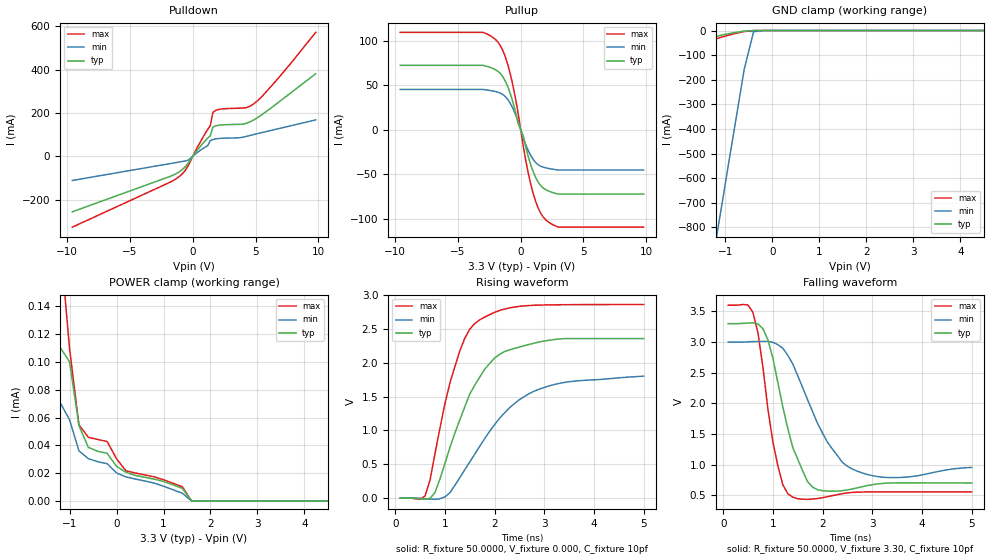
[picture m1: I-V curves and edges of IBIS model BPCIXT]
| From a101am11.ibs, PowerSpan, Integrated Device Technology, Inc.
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|   Model PCI tristate_driver
[Model]   BPCIXT
Model_type   I/O
Polarity   Non-Inverting
Enable   Active-High
Vinl = 1.16v
Vinh = 1.65v
C_comp   10.5pf   8pf   12pf
[Temperature Range]   27.0   125.0   -40.0
[Pullup Reference]   3.30V   3.00V   3.60V
[Pulldown Reference]   0.00V   0.00V   0.00V
[POWER Clamp Reference]   3.30V   3.00V   3.60V
[GND Clamp Reference]   0.00V   0.00V   0.00V
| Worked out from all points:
|   slope of the pulldown table from 0 to 0.495 V, typ, clamps not added: 13 ohm
|   slope of the pullup table from 0 to 0.495 V, typ, clamps not added: 20.4 ohm
|   GND clamp passes 1 mA (typ) near -0.47 V on its own axis
|   POWER clamp passes 1 mA (typ) near -2.20 V on its own axis
|   rising waveform, R_fixture 50.0000, V_fixture 0.000, C_fixture 10pf: 20-80 % time 802ps typ, 1.13ns min, 582ps max; typ from 0 V to 2.36 V
|   falling waveform, R_fixture 50.0000, V_fixture 3.30, C_fixture 10pf: 20-80 % time 446ps typ, 673ps min, 325ps max; typ from 3.3 V to 0.7 V
[Pulldown]
|   volt   I(typ)   I(min)   I(max)
-9.6V     -256.8mA   -112mA     -327.7mA
-1.8V     -93.12mA   -34mA      -119.8mA
-1V       -68.86mA   -26mA      -90.01mA
-400mV    -34.11mA   -19.2mA    -46.95mA
1.2V      84.05mA    49.29mA    125.1mA
1.4V      94.99mA    72.6mA     142.2mA
1.6V      134.1mA    76.97mA    201.7mA
2.2V      144.1mA    82.47mA    217.6mA
4.2V      150.9mA    90.54mA    223.7mA
5V        172.4mA    102.3mA    248.3mA
7V        256.6mA    129.6mA    372.8mA
9.8V      381.2mA    167.8mA    572.4mA
[Pullup]
|volt  I(typ)   I(min)   I(max)
-9.6V     72.37mA    45.28mA    109.5mA
-3V       72.37mA    45.28mA    109.5mA
-1.8V     65.55mA    42.08mA    98.22mA
-1.2V     53.9mA     36.95mA    80.94mA
-800mV    39.41mA    28.97mA    61.1mA
-400mV    19.13mA    16.72mA    34.19mA
400mV     -19.13mA   -16.72mA   -34.19mA
1V        -47.37mA   -33.48mA   -71.9mA
1.6V      -62.88mA   -41.03mA   -93.99mA
2.2V      -68.78mA   -43.48mA   -103.6mA
3V        -72.37mA   -45.28mA   -109.5mA
9.8V      -72.37mA   -45.28mA   -109.5mA
[GND_clamp]
|volt   I(typ)   I(min)   I(max)
-9.6V     -437.1mA   -10.59A    -530.5mA
-1.2V     -23.99mA   -851.9mA   -33.77mA
-1V       -15.53mA   -620mA     -22.63mA
-600mV    -2.506mA   -158.4mA   -4.199mA
-400mV    -152.4uA   -4.992mA   -240.4uA
-200mV    -18.8uA    -41.37uA   -20.15uA
9.8V      0A         0A         0A
[POWER_clamp]
|volt   I(typ)   I(min)   I(max)
-9.6V     375.8mA    141.4mA    680.3mA
-2V       218.9uA    142.9uA    294.9uA
-1.6V     163.9uA    96.81uA    197.2uA
-1.4V     145.2uA    92.55uA    191.4uA
-1.2V     110.5uA    70.81uA    187uA
-1V       100.1uA    58.5uA     109.7uA
-800mV    54.28uA    36.11uA    54.76uA
-600mV    38.64uA    30.54uA    45.9uA
-200mV    34.38uA    26.87uA    42.86uA
0V        25uA       20.28uA    30.44uA
1.6V      0A         0A         0A
9.8V      0A         0A         0A
[Ramp]
| variable   typ   min   max
dV/dt_r   1.42/0.80ns   1.08/1.10ns   1.72/0.60ns
dV/dt_f   1.99/0.50ns   1.81/0.80ns   2.17/0.30ns
R_load = 50.0000
[Rising Waveform]
R_fixture = 50.0000
V_fixture = 0.000
C_fixture = 10pf
| time   V(typ)   V(min)   V(max)
100ps     95.26uV    144.1uV    68.65uV
600ps     -17.91mV   -8.712mV   32.78mV
700ps     -2.232mV   -15.05mV   268.1mV
800ps     83.71mV    -17.81mV   660.1mV
1.1ns     749.9mV    79.77mV    1.704V
1.4ns     1.351V     421.1mV    2.365V
1.6ns     1.67V      650.6mV    2.583V
2.1ns     2.126V     1.181V     2.774V
2.8ns     2.292V     1.583V     2.852V
5ns       2.359V     1.803V     2.863V
[Falling Waveform]
R_fixture = 50.0000
V_fixture = 3.30
V_fixture_min = 3.00
V_fixture_max = 3.60
C_fixture = 10pf
| time   V(typ)   V(min)   V(max)
100ps     3.3V       3V         3.6V
600ps     3.313V     3.007V     3.48V
700ps     3.294V     3.009V     3.149V
900ps     3.038V     3.009V     1.908V
1.1ns     2.339V     2.957V     984.7mV
1.3ns     1.592V     2.784V     525.4mV
1.8ns     632.7mV    1.863V     438.6mV
2.5ns     586.5mV    972.9mV    538mV
3.4ns     700.3mV    788.3mV    555.5mV
5ns       700mV      954.7mV    555.7mV
